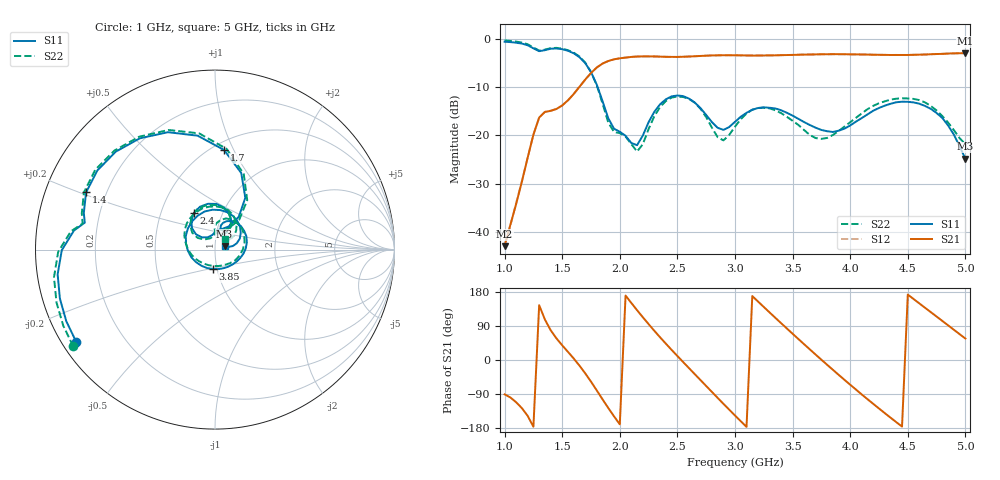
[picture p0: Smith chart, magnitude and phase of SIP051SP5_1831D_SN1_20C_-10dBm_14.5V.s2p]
# GHz  S  dB  R  50
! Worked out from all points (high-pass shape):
!   81 points, 1 GHz to 5 GHz, reference 50 ohm
!   highest |S21| = -3.01 dB at 5 GHz (marker M1); lowest = -42.9 dB at 1 GHz (marker M2)
!   |S21| within 3 dB of the highest: 1.798 GHz to end of sweep
!   lowest |S11| = -24.8 dB at 5 GHz (marker M3), VSWR 1.12, Z = 55.6 + j2.29 ohm
!   |S11| at or under -10 dB: 1.807 GHz to end of sweep
!   |S22| runs from -23.3 to -0.4 dB; largest |S21 - S12| = 0.0021
!   S11 on the Smith chart (normalised r, x): 1 GHz: 0.04, -0.30; 1.4 GHz: 0.13, +0.21; 1.7 GHz: 0.57, +0.92; 2.4 GHz: 0.73, +0.32; 3.85 GHz: 0.95, -0.21; 5 GHz: 1.11, +0.05
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1  -0.65 -146.4  -42.89 -90.7  -42.52 -89.2  -0.39 -145.6
1.3  -2.60 168.3  -16.31 144.7  -16.33 144.6  -2.48 168.8
1.4  -2.09 156.0  -14.93 78.5  -14.91 78.4  -1.97 156.4
1.55  -2.52 124.1  -12.75 21.4  -12.75 21.4  -2.41 123.9
1.7  -5.07 84.8  -8.47 -35.3  -8.49 -35.3  -4.96 83.5
1.85  -12.93 54.1  -5.16 -103.7  -5.16 -103.8  -13.40 51.0
2.05  -20.09 89.6  -3.93 170.0  -3.93 170.1  -20.24 87.3
2.2  -20.03 137.0  -3.68 112.8  -3.69 112.8  -21.83 135.9
2.35  -13.56 129.1  -3.73 59.8  -3.73 59.8  -14.14 135.2
2.4  -12.54 119.7  -3.77 43.0  -3.77 43.0  -12.90 124.8
2.55  -11.88 88.0  -3.75 -5.4  -3.76 -5.4  -12.07 90.7
2.75  -15.79 57.6  -3.54 -68.7  -3.53 -68.7  -16.23 55.1
3  -17.20 76.4  -3.45 -146.5  -3.44 -146.4  -18.19 91.4
3.2  -14.34 51.5  -3.50 154.3  -3.50 154.3  -14.36 60.5
3.4  -14.81 12.5  -3.43 97.3  -3.43 97.2  -15.40 14.0
3.7  -18.41 -52.8  -3.27 14.3  -3.27 14.3  -20.55 -77.0
3.85  -19.30 -96.9  -3.22 -25.9  -3.23 -26.0  -19.92 -130.2
4.1  -16.43 -177.3  -3.29 -90.9  -3.28 -90.8  -15.47 166.6
4.35  -13.48 117.3  -3.39 -152.2  -3.40 -152.1  -12.61 117.1
4.55  -13.19 72.1  -3.35 161.0  -3.36 160.9  -12.47 79.4
4.75  -15.38 32.7  -3.19 114.7  -3.19 114.6  -14.85 48.5
5  -24.83 21.0  -3.01 56.6  -3.01 56.6  -21.82 45.6
